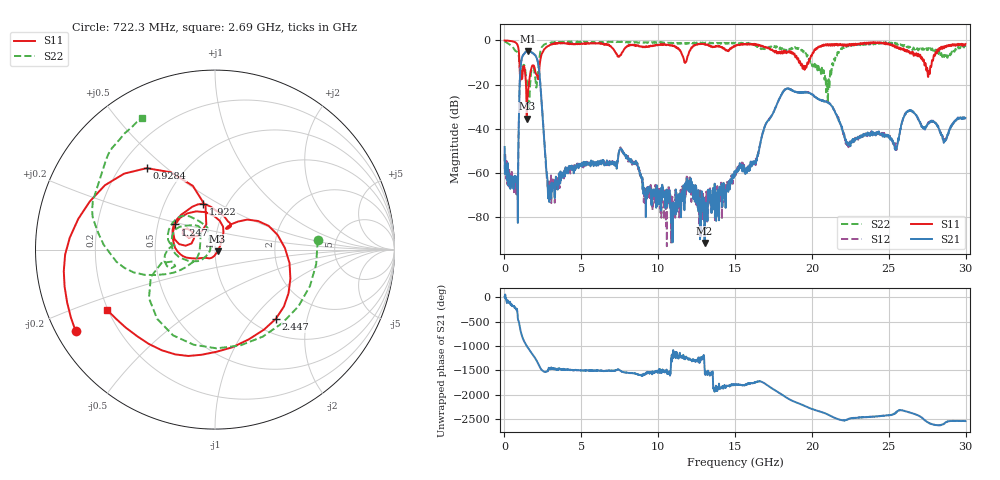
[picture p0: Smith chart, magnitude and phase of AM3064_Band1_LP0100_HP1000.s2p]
# Hz S DB R 50.0
!freq dBS11 angS11 dBS21 angS21 dBS12 angS12 dBS22 angS22
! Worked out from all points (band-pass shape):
!   1600 points, 10 MHz to 29.98 GHz, reference 50 ohm
!   highest |S21| = -4.74 dB at 1.528 GHz (marker M1); lowest = -91.8 dB at 13.02 GHz (marker M2)
!   |S21| within 3 dB of the highest: 1.147 GHz to 2.085 GHz (938.6 MHz wide, 58.1 % of centre)
!   lowest |S11| = -35.5 dB at 1.453 GHz (marker M3), VSWR 1.03, Z = 51.5 - j0.874 ohm
!   |S11| at or under -10 dB: 973.8 MHz to 2.311 GHz (1.337 GHz wide, 81.4 % of centre); 19.24 GHz to 19.71 GHz (468.2 MHz wide, 2.4 % of centre); 27.3 GHz to 27.8 GHz (497 MHz wide, 1.8 % of centre)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
!   |S22| runs from -31.1 to -0.4 dB; largest |S21 - S12| = 0.0079
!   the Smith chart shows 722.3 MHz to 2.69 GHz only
!   S11 on the Smith chart (normalised r, x): 722.3 MHz: 0.06, -0.27; 928.4 MHz: 0.31, +0.43; 1.247 GHz: 0.62, +0.19; 1.922 GHz: 0.77, +0.43; 2.447 GHz: 1.26, -1.32; 2.69 GHz: 0.20, -0.25
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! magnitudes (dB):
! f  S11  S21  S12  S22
! 10 MHz  0.0  -48.3  -51.7  -0.4
! 722.3 MHz  -0.9  -64.1  -66.5  -4.8
! 928.4 MHz  -4.5  -39.2  -39.3  -6.8
! 1.247 GHz  -11.6  -6.4  -6.3  -11.1
! 1.453 GHz  -35.5  -4.9  -4.8  -18.2
! 1.528 GHz  -23.7  -4.7  -4.7  -23.2
! 1.922 GHz  -11.5  -6.2  -6.1  -13.3
! 2.447 GHz  -5.8  -30.8  -30.8  -2.9
! 2.69 GHz  -3.2  -54.3  -56.3  -1.5
! 2.972 GHz  -2.0  -66.0  -65.5  -1.1
! 5.015 GHz  -1.4  -55.9  -55.6  -0.8
! 7.62 GHz  -5.8  -49.4  -49.3  -0.7
! 10 GHz  -2.0  -72.9  -73.6  -0.9
! 13.02 GHz  -1.9  -91.8  -72.0  -1.2
! 15 GHz  -2.6  -61.5  -60.5  -1.5
! 18.21 GHz  -5.6  -22.6  -22.5  -4.4
! 19.99 GHz  -6.9  -24.5  -24.3  -10.8
! 21.02 GHz  -1.7  -28.1  -28.2  -25.9
! 22.35 GHz  -2.0  -47.2  -46.4  -2.5
! 25 GHz  -1.4  -43.5  -43.7  -1.2
! 27.58 GHz  -14.7  -37.6  -37.0  -3.5
! 29.98 GHz  -1.7  -35.2  -35.4  -2.9
